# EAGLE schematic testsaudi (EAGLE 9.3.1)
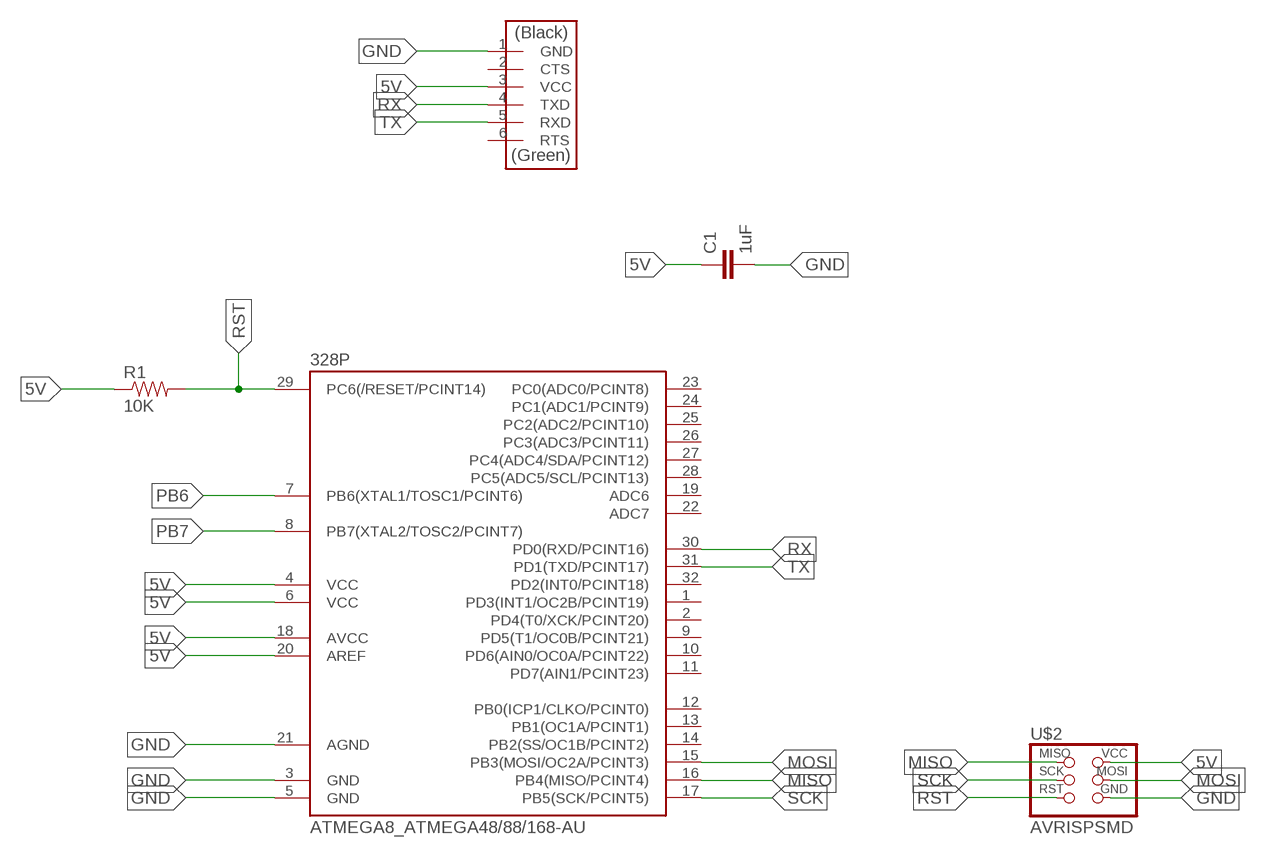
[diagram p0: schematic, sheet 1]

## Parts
328P  ATMEGA8_ATMEGA48/88/168-AU  [ATMEGA8_TQFP32-08]
C1  1uF  01_SPARKFUN_CAP1206  [01_SPARKFUN_1206]
R1  10K  01_SPARKFUN_RESISTOR1206  [01_SPARKFUN_1206]
U$1  FTDI-SMD-HEADER  [1X06SMD]
U$2  AVRISPSMD  [2X03SMD]

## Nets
5V: 328P.4(VCC) 328P.6(VCC) 328P.18(AVCC) 328P.20(AREF) C1.1 R1.1 U$1.3(VCC) U$2.2(VCC)
GND: 328P.3(GND) 328P.5(GND) 328P.21(AGND) C1.2 U$1.1(GND) U$2.6(GND)
MISO: 328P.16(PB4(MISO/PCINT4)) U$2.1(MISO)
MOSI: 328P.15(PB3(MOSI/OC2A/PCINT3)) U$2.4(MOSI)
PB6: 328P.7(PB6(XTAL1/TOSC1/PCINT6))
PB7: 328P.8(PB7(XTAL2/TOSC2/PCINT7))
RST: 328P.29(PC6(/RESET/PCINT14)) R1.2 U$2.5(RST)
RX: 328P.30(PD0(RXD/PCINT16)) U$1.4(TXD)
SCK: 328P.17(PB5(SCK/PCINT5)) U$2.3(SCK)
TX: 328P.31(PD1(TXD/PCINT17)) U$1.5(RXD)
Unconnected: 328P.1(PD3(INT1/OC2B/PCINT19)) 328P.2(PD4(T0/XCK/PCINT20)) 328P.9(PD5(T1/OC0B/PCINT21)) 328P.10(PD6(AIN0/OC0A/PCINT22)) 328P.11(PD7(AIN1/PCINT23)) 328P.12(PB0(ICP1/CLKO/PCINT0)) 328P.13(PB1(OC1A/PCINT1)) 328P.14(PB2(SS/OC1B/PCINT2)) 328P.19(ADC6) 328P.22(ADC7) 328P.23(PC0(ADC0/PCINT8)) 328P.24(PC1(ADC1/PCINT9)) 328P.25(PC2(ADC2/PCINT10)) 328P.26(PC3(ADC3/PCINT11)) 328P.27(PC4(ADC4/SDA/PCINT12)) 328P.28(PC5(ADC5/SCL/PCINT13)) 328P.32(PD2(INT0/PCINT18)) U$1.2(CTS) U$1.6(RTS)

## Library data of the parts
328P = satshakit_cnc:ATMEGA8_ATMEGA48/88/168
C1 = satshakit_cnc:01_SPARKFUN_CAP: Capacitor
R1 = satshakit_cnc:01_SPARKFUN_RESISTOR: Resistor
U$1 = fab:FTDI-SMD-HEADER
U$2 = fab:AVRISP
